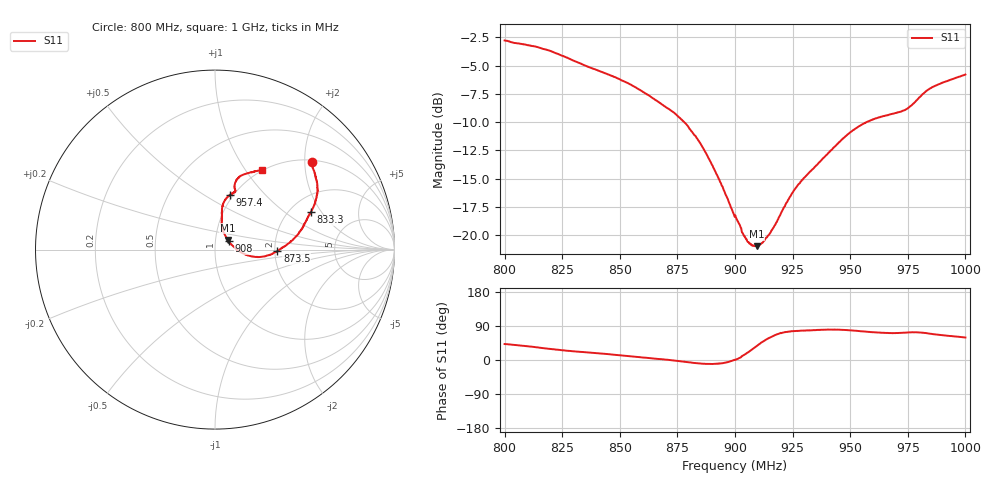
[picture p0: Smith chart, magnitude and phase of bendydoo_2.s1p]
# HZ S RI R 50
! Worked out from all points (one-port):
!   1010 points, 800 MHz to 1 GHz, reference 50 ohm
!   lowest |S11| = -21.0 dB at 909.4 MHz (marker M1), VSWR 1.20, Z = 57.3 + j6.19 ohm
!   |S11| at or under -10 dB: 877.9 MHz to 957.1 MHz (79.19 MHz wide, 8.63 % of centre)
!   S11 on the Smith chart (normalised r, x): 800 MHz: 1.05, +2.17; 833.3 MHz: 2.58, +1.60; 873.5 MHz: 2.07, -0.04; 908 MHz: 1.16, +0.11; 957.4 MHz: 0.97, +0.66; 1 GHz: 1.00, +1.20
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8e8  0.5394 0.4877
8.152626e8  0.57 0.3616
8.251734e8  0.5602 0.2697
8.333003e8  0.5345 0.208
8.501486e8  0.4769 0.1061
8.59663e8  0.4302 0.0513
8.735381e8  0.3479 -0.00815
8.751239e8  0.3364 -0.0137
8.794846e8  0.3028 -0.0298
8.866204e8  0.2344 -0.0413
8.929633e8  0.1749 -0.0283
9.000991e8  0.1224 0.000818
9.04658e8  0.0929 0.0272
9.06442e8  0.0841 0.037
9.080277e8  0.0772 0.0459
9.094152e8  0.0714 0.0535
9.11992e8  0.062 0.0686
9.153617e8  0.0516 0.0884
9.250743e8  0.0372 0.1499
9.316154e8  0.0375 0.1825
9.41328e8  0.04 0.2315
9.500495e8  0.058 0.279
9.573835e8  0.0846 0.3057
9.676907e8  0.1117 0.3242
9.750247e8  0.1092 0.348
9.795837e8  0.1189 0.3839
9.845391e8  0.1561 0.4167
9.999999e8  0.2626 0.4414
